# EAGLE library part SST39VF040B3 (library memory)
4 Mbit x8 Multi-Purpose Flash Source: http://www.sst.com/dotAsset/40782.pdf
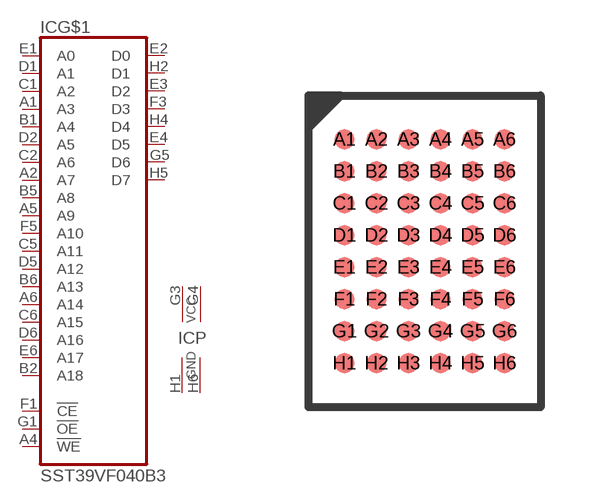
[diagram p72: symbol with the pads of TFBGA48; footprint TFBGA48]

Designator prefix IC; gates G$1=SST39VF040 P=PWRN2

## SST39VF040B3  [TFBGA48]
A1  G$1:A3  in
A2  G$1:A7  in
A4  G$1:!WE  in
A5  G$1:A9  in
A6  G$1:A14  in
B1  G$1:A4  in
B2  G$1:A18  in
B5  G$1:A8  in
B6  G$1:A13  in
C1  G$1:A2  in
C2  G$1:A6  in
C5  G$1:A11  in
C6  G$1:A15  in
D1  G$1:A1  in
D2  G$1:A5  in
D5  G$1:A12  in
D6  G$1:A16  in
E1  G$1:A0  in
E2  G$1:D0
E3  G$1:D2
E4  G$1:D5
E6  G$1:A17  in
F1  G$1:!CE  in
F3  G$1:D3
F5  G$1:A10  in
G1  G$1:!OE  in
G3  P:VCC  pwr
G4  P:VCC  pwr
G5  G$1:D6
H1  P:GND  pwr
H2  G$1:D1
H4  G$1:D4
H5  G$1:D7
H6  P:GND  pwr

## Footprint TFBGA48 (pad centres in mm)
48-ball Thin-profile, Fine-pitch Ball Grid Array (TFBGA) 6mm x 8mm SST Package Code: B3K Source: http://www.sst.com/dotAsset/40782.pdf
smd 0.5 x 0.5: A1 -2,2.8; A2 -1.2,2.8; A3 -0.4,2.8; A4 0.4,2.8; A5 1.2,2.8; A6 2,2.8; B1 -2,2; B2 -1.2,2; B3 -0.4,2; B4 0.4,2; B5 1.2,2; B6 2,2; C1 -2,1.2; C2 -1.2,1.2; C3 -0.4,1.2; C4 0.4,1.2; C5 1.2,1.2; C6 2,1.2; D1 -2,0.4; D2 -1.2,0.4; D3 -0.4,0.4; D4 0.4,0.4; D5 1.2,0.4; D6 2,0.4; E1 -2,-0.4; E2 -1.2,-0.4; E3 -0.4,-0.4; E4 0.4,-0.4; E5 1.2,-0.4; E6 2,-0.4; F1 -2,-1.2; F2 -1.2,-1.2; F3 -0.4,-1.2; F4 0.4,-1.2; F5 1.2,-1.2; F6 2,-1.2; G1 -2,-2; G2 -1.2,-2; G3 -0.4,-2; G4 0.4,-2; G5 1.2,-2; G6 2,-2; H1 -2,-2.8; H2 -1.2,-2.8; H3 -0.4,-2.8; H4 0.4,-2.8; H5 1.2,-2.8; H6 2,-2.8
